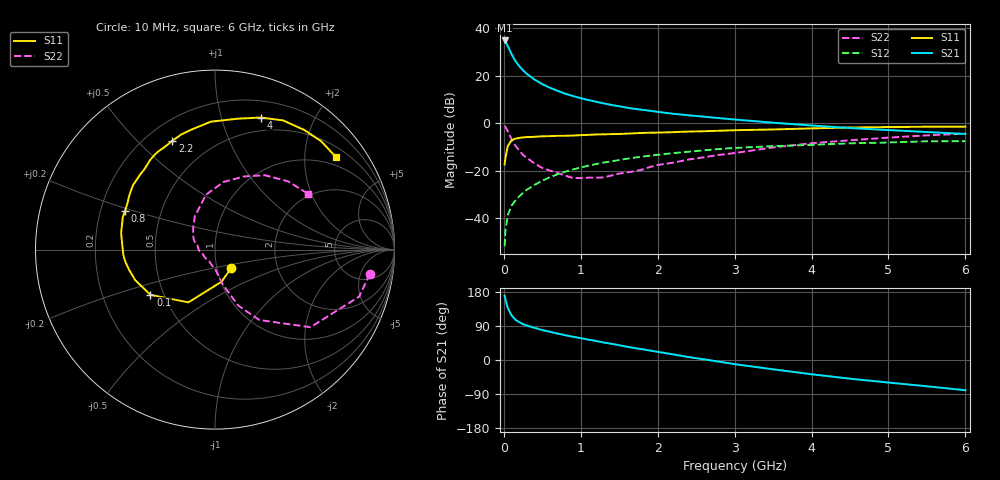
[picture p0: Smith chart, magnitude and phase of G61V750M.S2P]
! SIEMENS Small Signal Semiconductors
! BFG193
! Si NPN RF Bipolar Junction Transistor in SOT223
! VCE = 1.75 V  IC = 50 mA
! Common Emitter S-Parameters:  August  1996
# GHz  S  MA  R  50
!  f  S11  S21  S12  S22
! GHz  MAG  ANG  MAG  ANG  MAG  ANG  MAG  ANG
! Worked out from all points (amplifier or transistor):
!   36 points, 10 MHz to 6 GHz, reference 50 ohm
!   highest |S21| = 34.8 dB at 10 MHz (marker M1)
!   |S21| within 3 dB of that: start of sweep to 60.47 MHz
!   unconditionally stable (mu >= 1): 341.4 MHz to 2.626 GHz
!   at 250 MHz: K = 0.95, MSG = 25.7 dB, |S12| = -29.3 dB
!   at 1.4 GHz: K = 1.06, MAG = 10.3 dB, |S12| = -16.0 dB
!   at 6 GHz: K = 0.95, MSG = 1.5 dB, |S12| = -7.5 dB
!   S11 on the Smith chart (normalised r, x): 10 MHz: 1.17, -0.24; 100 MHz: 0.42, -0.26; 800 MHz: 0.31, +0.19; 2.2 GHz: 0.30, +0.64; 4 GHz: 0.36, +1.34; 6 GHz: 0.75, +2.76
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0.01  0.1364 -48.6  55.11 169.7  0.0026 80.1  0.8738 -8.9
0.02  0.1823 -78.2  52.73 160.6  0.0053 77.5  0.8443 -18.1
0.05  0.3294 -116.8  42.41 137.9  0.0116 67.8  0.6856 -39.1
0.1  0.4392 -145.0  28.46 117.9  0.0185 63.5  0.4635 -57.8
0.15  0.4757 -159.0  20.41 106.2  0.0237 63.9  0.338 -67.4
0.2  0.4913 -166.6  15.91 99.8  0.029 66.1  0.2666 -71.3
0.25  0.5047 -172.5  12.93 94.6  0.0344 66.5  0.2153 -75.5
0.3  0.5114 -176.7  10.9 90.8  0.04 67.7  0.1867 -78.4
0.4  0.5184 176.4  8.259 84.8  0.0507 67.9  0.1419 -83.4
0.5  0.5314 169.9  6.637 79.0  0.0621 66.7  0.1148 -87.8
0.6  0.5358 165.4  5.567 74.3  0.0734 65.7  0.101 -93.2
0.8  0.5451 156.7  4.175 65.4  0.0957 62.5  0.0787 -109.4
1.1  0.5703 145.5  3.07 53.8  0.128 56.9  0.0718 -138.4
1.3  0.5851 138.2  2.611 46.1  0.1494 52.6  0.0727 -160.8
1.6  0.6048 128.7  2.125 35.1  0.1793 45.5  0.0927 177.0
2.2  0.6504 111.5  1.584 14.9  0.2355 31.3  0.1483 145.3
2.8  0.6954 96.3  1.282 -4.5  0.2877 16.9  0.2161 121.5
3.5  0.7401 80.2  1.027 -24.6  0.3298 -0.9  0.3098 99.4
4  0.7791 70.8  0.898 -37.6  0.351 -10.8  0.38 82.8
4.5  0.8136 62.2  0.793 -49.3  0.3784 -20.9  0.4384 68.4
5.5  0.8455 45.6  0.654 -69.4  0.4173 -43.9  0.5567 43.1
6  0.8478 37.6  0.595 -79.8  0.4193 -57.0  0.6053 30.9
